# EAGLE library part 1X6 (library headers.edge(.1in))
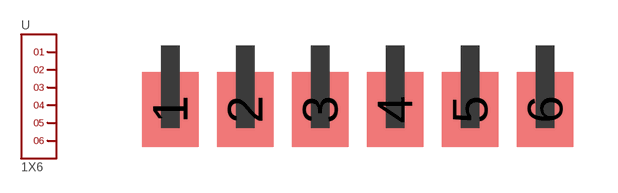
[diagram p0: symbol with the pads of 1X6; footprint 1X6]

Designator prefix -

## 1X6  [1X6]
1  1
2  2
3  3
4  4
5  5
6  6

## Footprint 1X6 (pad centres in mm)
smd 1.905 x 2.54: 1 0,-2.159; 2 2.54,-2.159; 3 5.08,-2.159; 4 7.62,-2.159; 5 10.16,-2.159; 6 12.7,-2.159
